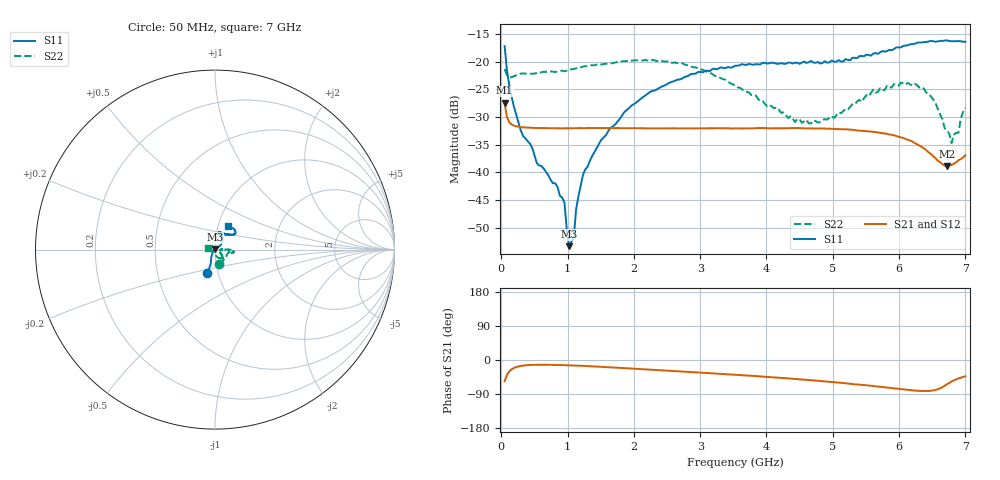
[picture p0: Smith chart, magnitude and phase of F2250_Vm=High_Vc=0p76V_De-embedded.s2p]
! Integrated Device Technology
! Corporate Headquarters
! 6024 Silver Creek Valley Road
! San Jose, CA 95138  USA
! Phone:  1-408-284-8200
! Toll Free:  1-800-223-1366
! Webpage:  http://www.idt.com/
! Timing and RF Division
! 515 Groton Road, Suite 102
! Westford, MA 01886-6024
! Device:  F2250
! Description: Voltage Variable RF Attenuator
! Frequency:  50.0 -  6000.00 MHz
! Package:  3x3 mm Thin QFN Plastic Package: 16 pin
! Ports:  2 RF, 3 DC
!  Pin  1  = GND
!  Pin  2  = NC
!  Pin  3  = RF1  = Port 1
!  Pin  4  = NC
!  Pin  5  = GND
!  Pin  6  = GND
!  Pin  7  = GND
!  Pin  8  = GND
!  Pin  9  = NC
!  Pin 10  = RF2  = Port 2
!  Pin 11  = NC
!  Pin 12  = GND
!  Pin 13  = GND
!  Pin 14  = VCNTRL
!  Pin 15  = VDD
!  Pin 16  = VMODE
! Vcntrl:  0.760 Volts
! Vmode:  +3.300 Volts
! Vdd:  +3.30  Volts
! Current:  1.298 mA
! Data:  The device was measured on a the F2250 evaluation board which has
!  individual transmission lines to the RF pins.  Data was collected
!  using a calibrated network analyzer.  The evaluation board was
!  de-embedded using a TRL calibration technique.
!  The reference plane is the edge of the package pin.
! Misc:  SN 10
!  Action Tracker AT0258
! Date Measured:  2014-11-26
! Date:  2015-10-15  MJV
! Note:
!  Integrated Device Technology supplies this data as a sample of measured
!  data at the package pin for this product.  Your particular data for this
!  product may vary.
!  Data was taken at 25 degrees C.
!  Integrated Device Technology reserves the right to change this data at anytime.
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# GHz S dB R 50
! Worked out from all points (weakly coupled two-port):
!   201 points, 50 MHz to 7 GHz, reference 50 ohm
!   highest |S21| = -27.41 dB at 50 MHz (marker M1); lowest = -38.8 dB at 6.722 GHz (marker M2)
!   lowest |S11| = -53.4 dB at 1.023 GHz (marker M3), VSWR 1.00, Z = 49.9 + j0.158 ohm
!   |S11| at or under -10 dB: start of sweep to end of sweep
!   |S22| runs from -34.7 to -19.6 dB; largest |S21 - S12| = 0.00012
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0.05  -17.15 -107.9  -27.41 -56.3  -27.41 -56.3  -21.29 -73.6
0.1195  -24.20 -111.1  -30.92 -30.4  -30.91 -30.4  -22.70 -25.8
0.29325  -32.39 -125.4  -31.81 -15.7  -31.81 -15.7  -22.13 -12.1
0.9535  -45.52 173.1  -32.02 -13.6  -32.04 -13.6  -21.71 -10.5
1.023  -53.37 132.3  -32.02 -14.0  -32.02 -14.0  -21.41 -10.4
1.0925  -51.91 70.7  -32.01 -14.4  -32.02 -14.4  -21.31 -10.4
1.12725  -46.85 50.7  -32.01 -14.7  -32.01 -14.7  -21.17 -10.9
1.2315  -40.47 36.1  -32.00 -15.4  -31.99 -15.5  -20.87 -11.9
1.6485  -31.93 39.3  -31.98 -19.3  -31.99 -19.3  -20.30 -10.6
2.37825  -24.75 45.8  -32.02 -26.8  -32.02 -26.8  -19.76 -7.0
3.525  -20.70 71.3  -32.05 -39.0  -32.04 -39.0  -24.31 -0.4
4.4285  -20.16 74.4  -31.99 -49.9  -31.99 -50.0  -30.90 -4.1
4.7065  -20.13 71.7  -32.05 -53.8  -32.05 -53.9  -30.61 -14.6
5.01925  -19.96 63.1  -32.14 -58.8  -32.15 -58.8  -30.15 -24.5
5.61  -18.51 44.0  -32.66 -68.6  -32.64 -68.8  -25.02 -39.3
5.85325  -17.82 40.3  -33.15 -73.4  -33.14 -73.5  -24.58 -44.0
6.33975  -16.50 40.5  -35.40 -81.7  -35.41 -81.8  -24.53 -58.6
6.54825  -16.37 44.4  -37.45 -79.0  -37.43 -79.2  -27.36 -74.7
6.722  -16.13 49.1  -38.83 -63.9  -38.81 -63.9  -32.39 -110.0
6.7915  -16.28 51.1  -38.69 -56.4  -38.67 -56.5  -34.68 -134.1
6.89575  -16.25 56.2  -37.81 -48.7  -37.80 -48.7  -32.83 -174.8
7  -16.37 62.2  -36.91 -43.0  -36.90 -43.0  -28.34 164.8
